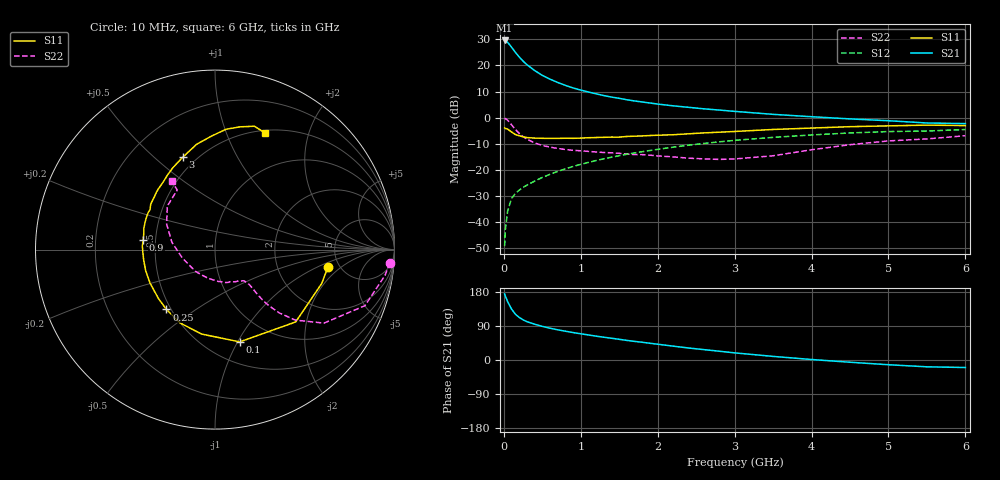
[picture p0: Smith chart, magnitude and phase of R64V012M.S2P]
! SIEMENS Small Signal Semiconductors
! BFR193
! Si NPN RF Bipolar Junction Transistor in SOT23
! VCE = 4 V  IC = 12 mA
! Common Emitter S-Parameters:  May  1996
# GHz  S  MA  R  50
!  f  S11  S21  S12  S22
! GHz  MAG  ANG  MAG  ANG  MAG  ANG  MAG  ANG
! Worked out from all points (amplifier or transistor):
!   36 points, 10 MHz to 6 GHz, reference 50 ohm
!   highest |S21| = 29.5 dB at 10 MHz (marker M1)
!   |S21| within 3 dB of that: start of sweep to 111.4 MHz
!   unconditionally stable (mu >= 1): 692 MHz to 1.994 GHz
!   at 250 MHz: K = 0.70, MSG = 24.1 dB, |S12| = -26.7 dB
!   at 1.4 GHz: K = 1.03, MAG = 10.4 dB, |S12| = -15.1 dB
!   at 6 GHz: K = 0.95, MSG = 1.1 dB, |S12| = -4.5 dB
!   S11 on the Smith chart (normalised r, x): 10 MHz: 4.02, -1.34; 100 MHz: 0.71, -1.02; 250 MHz: 0.47, -0.39; 900 MHz: 0.43, +0.06; 3 GHz: 0.42, +0.62; 6 GHz: 0.53, +1.38
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0.01  0.6362 -9.0  29.96 174.4  0.0035 87.4  0.9777 -4.3
0.02  0.6239 -17.6  29.79 168.6  0.0073 83.3  0.9582 -8.6
0.05  0.6037 -41.9  27.54 153.6  0.0166 73.0  0.892 -20.5
0.1  0.5322 -75.0  22.34 134.4  0.0285 63.1  0.7323 -34.0
0.15  0.4765 -99.0  17.79 120.8  0.0358 58.5  0.595 -41.3
0.2  0.4525 -115.7  14.48 112.4  0.0412 57.6  0.5018 -44.6
0.25  0.4294 -129.0  12.07 106.0  0.0465 57.6  0.4355 -46.1
0.3  0.4169 -139.0  10.32 101.2  0.0514 58.5  0.3888 -46.7
0.4  0.4072 -152.8  7.975 94.5  0.0613 60.5  0.3297 -46.4
0.5  0.4038 -162.9  6.446 88.7  0.0721 62.1  0.2949 -45.8
0.6  0.4016 -171.3  5.449 83.9  0.0828 63.2  0.2734 -45.6
0.7  0.4024 -177.9  4.717 79.7  0.0938 64.3  0.2584 -45.9
0.9  0.4037 172.0  3.707 72.4  0.1168 64.4  0.2381 -47.1
1.1  0.4139 163.2  3.096 66.1  0.1399 64.0  0.227 -50.5
1.3  0.4217 155.3  2.647 60.1  0.1639 62.9  0.216 -54.2
1.6  0.438 144.9  2.203 51.7  0.2002 60.6  0.2021 -62.4
2.2  0.4721 128.3  1.686 36.6  0.2733 54.0  0.1781 -84.3
3  0.5453 109.2  1.321 18.8  0.3692 43.0  0.1627 -131.6
3.5  0.5957 99.9  1.159 9.5  0.4205 35.5  0.1872 -164.9
4.5  0.6736 84.7  0.948 -5.9  0.5111 20.8  0.305 152.1
5.5  0.7215 72.3  0.792 -18.0  0.5563 5.6  0.3929 122.4
6  0.7076 66.8  0.771 -19.8  0.594 1.2  0.4522 122.2
